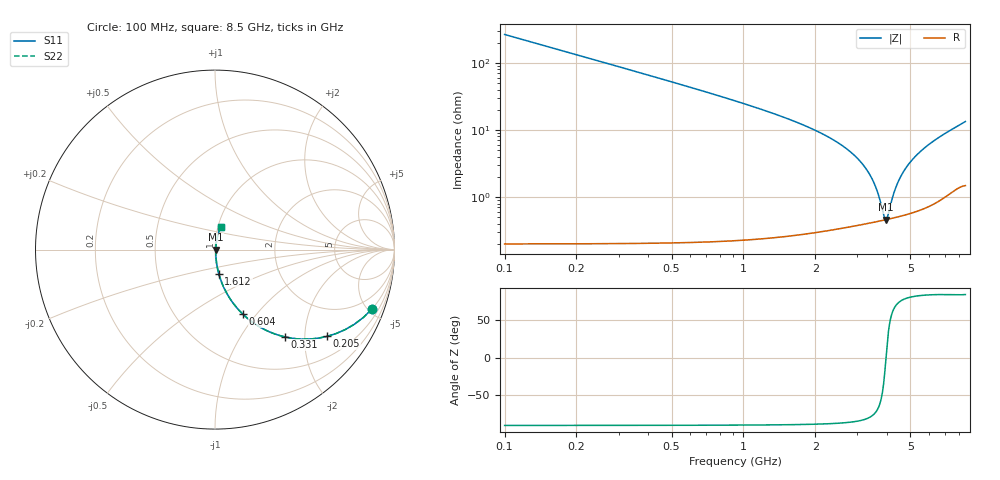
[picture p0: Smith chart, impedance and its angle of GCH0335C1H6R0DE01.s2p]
!Murata Part Number: GCH0335C1H6R0DE01
!These Parameters are Measured in Series Mode Connection
!Data Generated on Mar 13, 2026
!  o--ll--o
!Port1  Port2
!  o------o
!Operation Temp=25[degC], DC Bias Voltage=0[V]
!Freq. Start=100[MHz] Stop=9[GHz] 401[Steps]
# Hz S RI R 50
!Freq.(Hz) S11(Real) S11(Imag) S21(Real) S21(Imag) S12(Real) S12(Imag) S22(Real) S22(Imag)
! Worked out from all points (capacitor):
!   401 points, 100 MHz to 8.5 GHz, reference 50 ohm
!   read as one part in series: C = 6 pF near 142 MHz
!   lowest |Z| = 461 mohm at 3.943 GHz (marker M1)
!   series resonance near 3.953 GHz, so ESL is about 270 pH
!   S11 on the Smith chart (normalised r, x): 100 MHz: 1.00, -5.30; 205 MHz: 1.00, -2.58; 331 MHz: 1.00, -1.59; 604 MHz: 1.00, -0.86; 1.612 GHz: 1.01, -0.27; 8.5 GHz: 1.03, +0.27
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1e8  0.8752 -0.3301  0.1248 0.3301  0.1248 0.3301  0.8752 -0.3301
2.05e8  0.6246 -0.4834  0.3754 0.4834  0.3754 0.4834  0.6246 -0.4834
3.31e8  0.388 -0.486  0.612 0.486  0.612 0.486  0.388 -0.486
4.57e8  0.2477 -0.4299  0.7523 0.4299  0.7523 0.4299  0.2477 -0.4299
6.04e8  0.1566 -0.361  0.8434 0.361  0.8434 0.361  0.1566 -0.361
9.4e8  0.068 -0.2475  0.932 0.2475  0.932 0.2475  0.068 -0.2475
1.507e9  0.0245 -0.1464  0.9755 0.1464  0.9755 0.1464  0.0245 -0.1464
1.612e9  0.021 -0.134  0.979 0.134  0.979 0.134  0.021 -0.134
2.914e9  0.0054 -0.0414  0.9946 0.0414  0.9946 0.0414  0.0054 -0.0414
3.229e9  0.0047 -0.0273  0.9953 0.0273  0.9953 0.0273  0.0047 -0.0273
3.481e9  0.00446 -0.0171  0.9955 0.0171  0.9955 0.0171  0.00446 -0.0171
3.67e9  0.00443 -0.01  0.9956 0.01  0.9956 0.01  0.00443 -0.01
3.88e9  0.00452 -0.00252  0.9955 0.00252  0.9955 0.00252  0.00452 -0.00252
3.943e9  0.00457 -0.000349  0.9954 0.000349  0.9954 0.000349  0.00457 -0.000349
4.027e9  0.00466 0.0025  0.9953 -0.0025  0.9953 -0.0025  0.00466 0.0025
4.3e9  0.00504 0.0114  0.995 -0.0114  0.995 -0.0114  0.00504 0.0114
4.531e9  0.00549 0.0186  0.9945 -0.0186  0.9945 -0.0186  0.00549 0.0186
4.825e9  0.00621 0.0274  0.9938 -0.0274  0.9938 -0.0274  0.00621 0.0274
5.224e9  0.00746 0.0388  0.9925 -0.0388  0.9925 -0.0388  0.00746 0.0388
5.707e9  0.00941 0.0521  0.9906 -0.0521  0.9906 -0.0521  0.00941 0.0521
7.114e9  0.0184 0.0891  0.9816 -0.0891  0.9816 -0.0891  0.0184 0.0891
8.5e9  0.0312 0.1267  0.9688 -0.1267  0.9688 -0.1267  0.0312 0.1267
